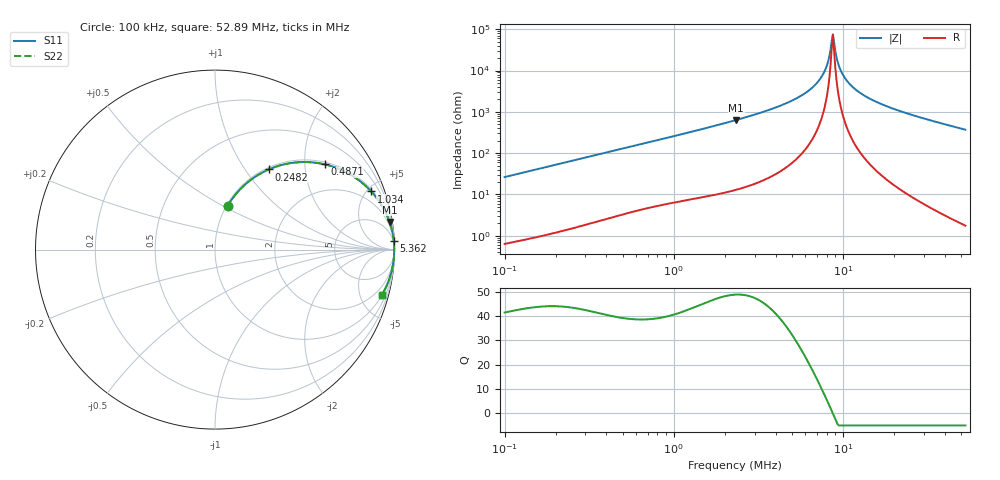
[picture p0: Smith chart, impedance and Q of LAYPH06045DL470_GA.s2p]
! LAYPH06045DL470_GA  S-PARAMETER MODEL  ( General Type )
! Model Generated by TAIYO YUDEN Corporation (http://www.ty-top.com)
! Version 2.0
! TAIYO YUDEN Control No. 180914NI43SB-FBB
! Copyright(c) 2018 TAIYO YUDEN CO.,LTD. All Rights Reserved.
! Product Description (link to TY-COMPAS)
! https://ds.yuden.co.jp/TYCOMPAS/or/detail?pn=LAYPH06045DL470MGA&u=M
! Products Name : Inductors
! Characteristics :
!  Inductance : 47 uH , SRF(min) : -Hz , DC Resistance(max) : 0.162 Ohm
!  Rated Current : Saturation :0.85 A , Temp Rise : 0.86 A (25 degC)
!  Case Size : 6.3 x 6.0 / 0.248 x 0.236 [mm/inch] , Thickness : 4.5 / 0.177 [mm/inch]
!  (Conditions: Temperature = 25 degC , DC Bias Current/Voltage = 0A / 0V)
! External Node Assignments :
!  1  o---GGG---o  2
! GND o---------o GND
! Frequency Range : 0.1MHz  -  52.890102MHz  [ 402 STEP ]
# MHz S RI R 50
! Freq[MHz].  S11 Real  S11 Imag  S21 Real  S21 Imag  S12 Real  S12 Imag  S22 Real  S22 Imag
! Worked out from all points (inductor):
!   401 points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, 100 kHz to 52.89 MHz, reference 50 ohm
!   read as one part in series: L = 41.7 uH near 103.2 kHz
!   highest Q = 48.9 at 2.336 MHz (marker M1), where L = 43.1 uH
!   self-resonance near 8.582 MHz
!   S11 on the Smith chart (normalised r, x): 100 kHz: 1.01, +0.53; 248.2 kHz: 1.03, +1.29; 487.1 kHz: 1.06, +2.52; 1.034 MHz: 1.13, +5.32; 5.362 MHz: 2, +43; 52.89 MHz: 1.04, -7.38
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0.1  0.0697 0.2429  0.9303 -0.2429  0.9303 -0.2429  0.0697 0.2429
0.24825  0.2988 0.4464  0.7012 -0.4464  0.7012 -0.4464  0.2988 0.4464
0.285868  0.3589 0.4681  0.6411 -0.4681  0.6411 -0.4681  0.3589 0.4681
0.487138  0.6101 0.4752  0.3899 -0.4752  0.3899 -0.4752  0.6101 0.4752
0.817204  0.8092 0.3804  0.1908 -0.3804  0.1908 -0.3804  0.8092 0.3804
1.033849  0.8703 0.324  0.1297 -0.324  0.1297 -0.324  0.8703 0.324
2.299785  0.9717 0.1558  0.0283 -0.1558  0.0283 -0.1558  0.9717 0.1558
2.336123  0.9726 0.1532  0.0274 -0.1532  0.0274 -0.1532  0.9726 0.1532
3.85803  0.9912 0.0821  0.00877 -0.0821  0.00877 -0.0821  0.9912 0.0821
5.362197  0.9963 0.0459  0.00371 -0.0459  0.00371 -0.0459  0.9963 0.0459
6.574344  0.9979 0.026  0.00213 -0.026  0.00213 -0.026  0.9979 0.026
7.690185  0.9985 0.0114  0.00151 -0.0114  0.00151 -0.0114  0.9985 0.0114
8.060502  0.9986 0.00707  0.00141 -0.00707  0.00141 -0.00707  0.9986 0.00707
8.582145  0.9987 0.00133  0.00134 -0.00133  0.00134 -0.00133  0.9987 0.00133
8.717747  0.9987 -0.000105  0.00134 0.000105  0.00134 0.000105  0.9987 -0.000105
8.855492  0.9987 -0.00154  0.00133 0.00154  0.00133 0.00154  0.9987 -0.00154
9.281924  0.9986 -0.00584  0.00135 0.00584  0.00135 0.00584  0.9986 -0.00584
9.57756  0.9986 -0.00872  0.00139 0.00872  0.00139 0.00872  0.9986 -0.00872
10.85731  0.9983 -0.0203  0.00169 0.0203  0.00169 0.0203  0.9983 -0.0203
13.52199  0.997 -0.0415  0.00297 0.0415  0.00297 0.0415  0.997 -0.0415
18.79393  0.9928 -0.077  0.0072 0.077  0.0072 0.077  0.9928 -0.077
52.8901  0.9306 -0.2517  0.0694 0.2517  0.0694 0.2517  0.9306 -0.2517
